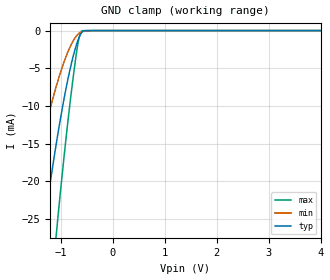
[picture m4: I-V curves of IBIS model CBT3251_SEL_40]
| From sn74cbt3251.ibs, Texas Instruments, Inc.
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[Model]   CBT3251_SEL_40
Model_type  Input
Vinl=0.8
Vinh=2.0
| variable   typ   min   max
C_comp   3.22pF   2.52pF   6.29pF
[Temperature Range]   40   100   -40
| Ambient temperature   25   85   -40
[Voltage range]   4   4   4
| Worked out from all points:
|   GND clamp passes 1 mA (typ) near -0.65 V on its own axis
[GND Clamp]
| CBT3251_SEL_40
|   Voltage   I(typ)   I(min)   I(max)
-4V       -193.4mA   -125.3mA   -297.5mA
-1.75V    -48.76mA   -27.7mA    -81.33mA
-1.7V     -45.95mA   -25.93mA   -76.95mA
-1.35V    -27.36mA   -14.53mA   -47.45mA
-1.31V    -25.38mA   -13.36mA   -44.25mA
-1.09V    -15.24mA   -7.519mA   -27.45mA
-1.07V    -14.39mA   -7.046mA   -26mA
-900mV    -7.787mA   -3.506mA   -14.48mA
-750mV    -3.158mA   -1.259mA   -5.703mA
-660mV    -1.157mA   -431.3uA   -1.426mA
-595mV    -251.3uA   -151.7uA   -36uA
4V        121.4pA    226.6pA    114.8pA
